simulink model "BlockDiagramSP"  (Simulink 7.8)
settings: Solver=ode45  StartTime=0.0  StopTime=10.0  RelTol=1e-3
undefined symbols (not defined in the file or in its folder): Ysp

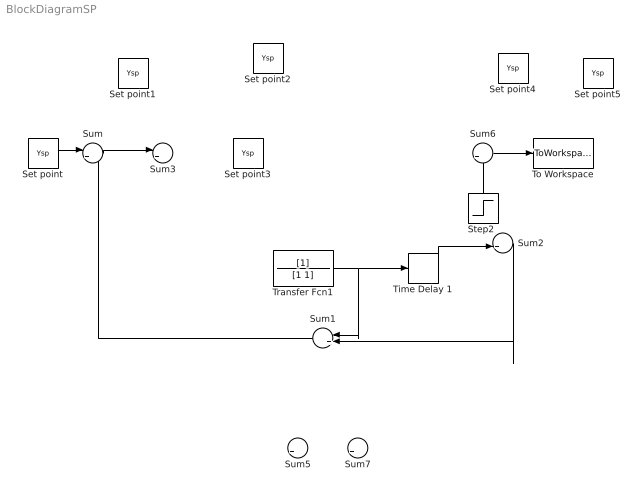
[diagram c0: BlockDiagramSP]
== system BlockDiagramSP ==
  Set point{,1..5} (6 alike) : Constant  Value=Ysp
  Step2 : Step  Time=0  SampleTime=0
  Sum : Sum  Inputs=|+-
  Sum{1,3,5..7} (5 alike) : Sum  Inputs=|++
  Sum2 : Sum  Inputs=|+-
  Time Delay 1 : TransportDelay
  To Workspace : ToWorkspace  VariableName=Y  SampleTime=-1  SaveFormat=Array
  Transfer Fcn1 : TransferFcn  Denominator=[1 1]
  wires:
  Set point/1 -> Sum/1
  Sum/1 -> Sum3/1
  ? -> ?
  Transfer Fcn1/1 -> Time Delay 1/1, Sum1/1
  Time Delay 1/1 -> Sum2/2
  Sum2/1 -> Sum1/2
  Sum1/1 -> Sum/2
  ? -> Sum6/1, Sum2/1
  Sum6/1 -> To Workspace/1
  Step2/1 -> Sum6/2
